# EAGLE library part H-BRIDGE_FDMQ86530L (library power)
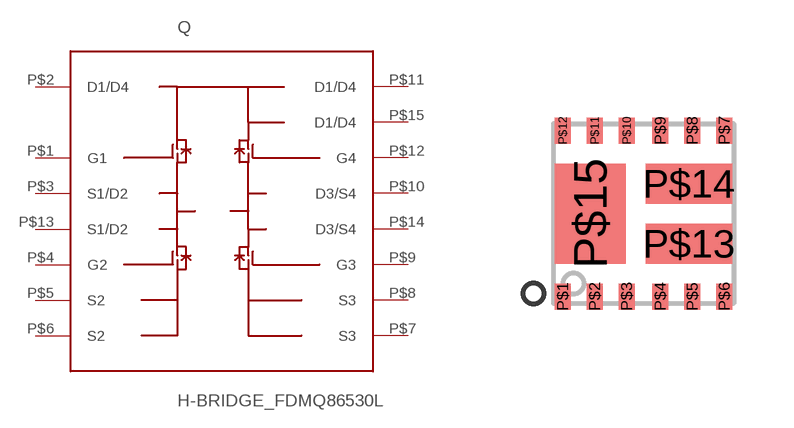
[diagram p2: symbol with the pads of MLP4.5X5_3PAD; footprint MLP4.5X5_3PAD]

Designator prefix Q

## H-BRIDGE_FDMQ86530L  [MLP4.5X5_3PAD]
P$1  G1
P$2  D1/D4
P$3  S1/D2
P$4  G2
P$5  S2
P$6  S2
P$7  S3
P$8  S3
P$9  G3
P$10  D3/S4
P$11  D1/D4
P$12  G4
P$13  S1/D2
P$14  D3/S4
P$15  D1/D4

## Footprint MLP4.5X5_3PAD (pad centres in mm)
smd 0.4 x 0.65: P$1 -2.02,-2.075; P$2 -1.22,-2.075; P$3 -0.42,-2.075; P$4 0.42,-2.075; P$5 1.22,-2.075; P$6 2.02,-2.075; P$7 2.02,2.075; P$8 1.22,2.075; P$9 0.42,2.075; P$10 -0.42,2.075; P$11 -1.22,2.075; P$12 -2.02,2.075
smd 2.17 x 1: P$13 1.135,-0.75; P$14 1.135,0.75
smd 1.78 x 2.5: P$15 -1.33,0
